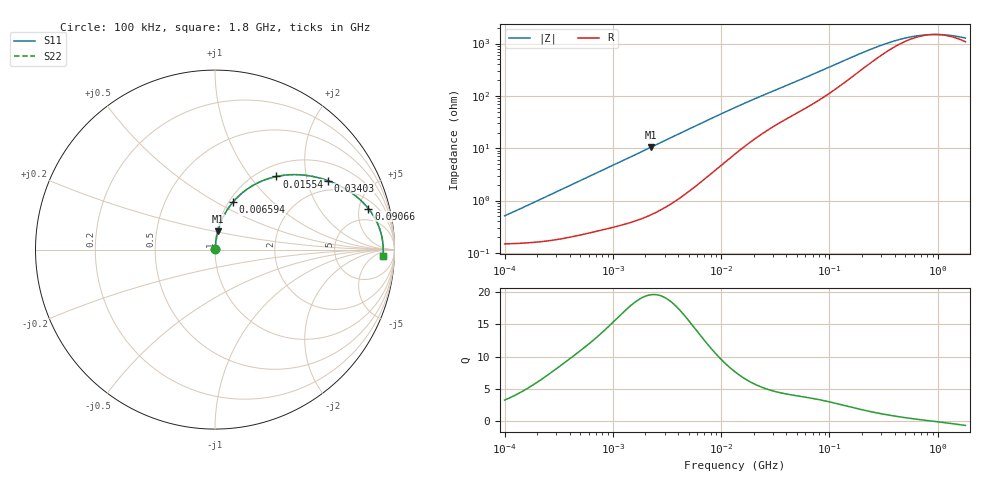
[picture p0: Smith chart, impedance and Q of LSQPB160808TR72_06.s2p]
! LSQPB160808TR72_06  S-PARAMETER MODEL  ( General Type )
! Model Generated by TAIYO YUDEN Corporation (http://www.ty-top.com)
! Version 1.0
! TAIYO YUDEN Control No. 110726NG25SE-FKC
! Copyright(c) 2011 TAIYO YUDEN CO.,LTD. All Rights Reserved.
! Product Description (link to TY-COMPAS)
! https://ds.yuden.co.jp/TYCOMPAS/or/detail?pn=LSQPB160808TR72M06&u=M
! Products Name : Inductors
! Characteristics :
!  Inductance : 0.72 uH , SRF(min) : 600 MHz , DC Resistance(max) : 0.1872 Ohm
!  Rated Current : Saturation :1000 mA , Temp Rise : 810 mA (40 degC)
!  Case Size : 1.6 x 0.8 / 0.063 x 0.031 [mm/inch] , Thickness : 0.8 / 0.031 [mm/inch]
!  (Conditions: Temperature = 25 degC , DC Bias Current/Voltage = 0A / 0V)
! External Node Assignments :
!  1  o---GGG---o  2
! GND o---------o GND
! Frequency Range : 0.1MHz  -  1800MHz  [ 402 STEP ]
# MHz S RI R 50
! Freq[MHz].  S11 Real  S11 Imag  S21 Real  S21 Imag  S12 Real  S12 Imag  S22 Real  S22 Imag
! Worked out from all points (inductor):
!   401 points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, 100 kHz to 1.8 GHz, reference 50 ohm
!   read as one part in series: L = 778 nH near 105 kHz
!   highest Q = 19.5 at 2.244 MHz (marker M1), where L = 740 nH
!   self-resonance near 939.6 MHz
!   S11 on the Smith chart (normalised r, x): 100 kHz: 1.00, +0.01; 6.594 MHz: 1.05, +0.60; 15.54 MHz: 1.20, +1.36; 34.03 MHz: 1.60, +2.69; 90.66 MHz: 2.96, +6.23; 1.8 GHz: 23, -13
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0.1  0.00151 0.00488  0.9985 -0.00488  0.9985 -0.00488  0.00151 0.00488
0.140908  0.00157 0.00687  0.9984 -0.00687  0.9984 -0.00687  0.00157 0.00687
0.516129  0.00283 0.0246  0.9972 -0.0246  0.9972 -0.0246  0.00283 0.0246
1.158292  0.00624 0.0539  0.9938 -0.0539  0.9938 -0.0539  0.00624 0.0539
2.244135  0.0159 0.1022  0.9841 -0.1022  0.9841 -0.1022  0.0159 0.1022
2.66389  0.0211 0.1203  0.9789 -0.1203  0.9789 -0.1203  0.0211 0.1203
4.347904  0.0493 0.1887  0.9507 -0.1887  0.9507 -0.1887  0.0493 0.1887
6.593697  0.1012 0.2657  0.8988 -0.2657  0.8988 -0.2657  0.1012 0.2657
9.291023  0.175 0.3337  0.825 -0.3337  0.825 -0.3337  0.175 0.3337
13.41641  0.2891 0.3927  0.7109 -0.3927  0.7109 -0.3927  0.2891 0.3927
15.54051  0.3426 0.4074  0.6574 -0.4074  0.6574 -0.4074  0.3426 0.4074
22.44079  0.4821 0.4162  0.5179 -0.4162  0.5179 -0.4162  0.4821 0.4162
34.03197  0.6279 0.3845  0.3721 -0.3845  0.3721 -0.3845  0.6279 0.3845
49.1428  0.734 0.3337  0.266 -0.3337  0.266 -0.3337  0.734 0.3337
69.24595  0.8106 0.276  0.1894 -0.276  0.1894 -0.276  0.8106 0.276
90.65972  0.8546 0.2287  0.1454 -0.2287  0.1454 -0.2287  0.8546 0.2287
163.204  0.9091 0.1376  0.0909 -0.1376  0.0909 -0.1376  0.9091 0.1376
357.3983  0.9323 0.0577  0.0677 -0.0577  0.0677 -0.0577  0.9323 0.0577
542.0029  0.9358 0.0299  0.0642 -0.0299  0.0642 -0.0299  0.9358 0.0299
802.0705  0.9371 0.00823  0.0629 -0.00823  0.0629 -0.00823  0.9371 0.00823
1186.925  0.9372 -0.0122  0.0628 0.0122  0.0628 0.0122  0.9372 -0.0122
1800  0.936 -0.0361  0.064 0.0361  0.064 0.0361  0.936 -0.0361
